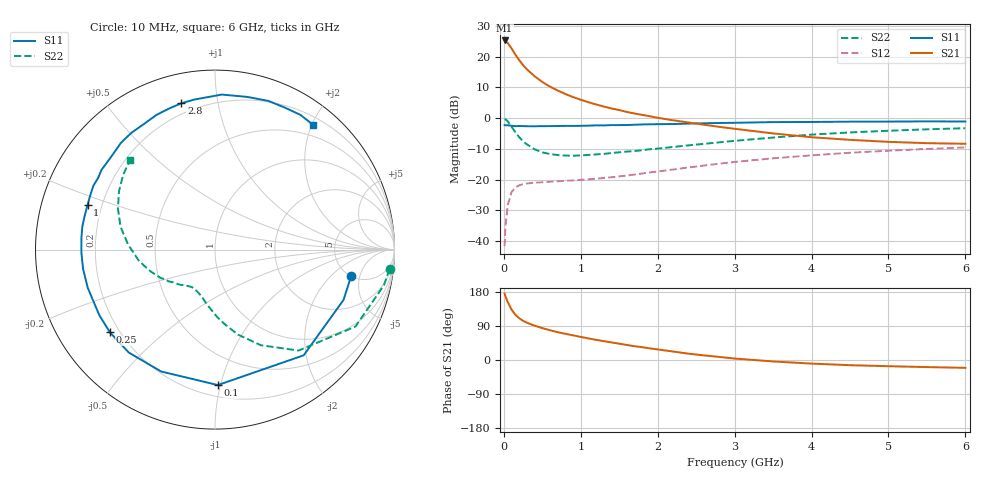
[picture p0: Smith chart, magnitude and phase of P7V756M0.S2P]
! SIEMENS Small Signal Semiconductors
! BFP196
! Si NPN RF Bipolar Junction Transistor in SOT143
! VCE = 0.75 V  IC = 6 mA
! Common Emitter S-Parameters:  May  1996
# GHz  S  MA  R  50
!  f  S11  S21  S12  S22
! GHz  MAG  ANG  MAG  ANG  MAG  ANG  MAG  ANG
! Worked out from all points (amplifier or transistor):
!   36 points, 10 MHz to 6 GHz, reference 50 ohm
!   highest |S21| = 25.3 dB at 10 MHz (marker M1)
!   |S21| within 3 dB of that: start of sweep to 110.3 MHz
!   unconditionally stable (mu >= 1): 1 GHz to end of sweep
!   at 250 MHz: K = 0.29, MSG = 19.4 dB, |S12| = -21.5 dB
!   at 1.4 GHz: K = 1.16, MAG = 8.7 dB, |S12| = -19.2 dB
!   at 6 GHz: K = 1.05, MAG = -0.7 dB, |S12| = -9.5 dB
!   S11 on the Smith chart (normalised r, x): 10 MHz: 5.07, -3.69; 100 MHz: 0.28, -0.98; 250 MHz: 0.16, -0.34; 1 GHz: 0.15, +0.17; 2.8 GHz: 0.14, +0.79; 6 GHz: 0.32, +2.01
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0.01  0.7732 -10.9  18.41 175.3  0.0083 84.4  0.9784 -6.3
0.02  0.769 -21.4  17.99 168.5  0.0165 79.7  0.962 -11.9
0.05  0.7688 -50.0  16.78 153.2  0.0386 65.3  0.8924 -28.7
0.1  0.7549 -88.8  13.68 133.1  0.063 48.2  0.7301 -50.4
0.15  0.7424 -113.8  10.8 119.4  0.0749 37.7  0.5906 -64.4
0.2  0.7482 -129.9  8.826 110.3  0.081 31.4  0.4912 -74.8
0.25  0.7451 -141.8  7.288 103.4  0.0845 27.3  0.4206 -82.4
0.3  0.741 -150.5  6.233 98.3  0.087 24.9  0.3758 -88.2
0.4  0.7402 -163.3  4.818 90.6  0.0893 22.3  0.3124 -97.6
0.5  0.7429 -171.6  3.881 84.2  0.0909 21.1  0.2787 -104.3
0.6  0.7446 -178.7  3.262 78.6  0.0927 20.7  0.2612 -109.4
0.7  0.7471 174.9  2.823 73.4  0.0943 21.3  0.2521 -113.9
0.8  0.7503 170.2  2.476 69.2  0.0957 21.7  0.2472 -117.9
1  0.7527 160.6  1.995 60.9  0.0994 24.0  0.2484 -123.9
1.1  0.758 156.4  1.82 56.9  0.1015 25.3  0.253 -126.7
1.6  0.776 138.3  1.263 39.6  0.1172 30.7  0.2867 -138.7
2.2  0.804 119.5  0.926 22.4  0.1465 33.7  0.3408 -152.4
2.8  0.8365 102.9  0.724 8.1  0.1821 31.9  0.4054 -167.3
3.5  0.8647 87.5  0.566 -3.8  0.2229 25.7  0.4849 176.7
4.5  0.88 70.3  0.445 -13.7  0.2747 15.0  0.5876 157.0
5.5  0.8888 57.6  0.393 -18.7  0.3167 3.7  0.6603 140.8
6  0.8842 51.9  0.384 -20.7  0.3351 -2.6  0.6884 133.3
